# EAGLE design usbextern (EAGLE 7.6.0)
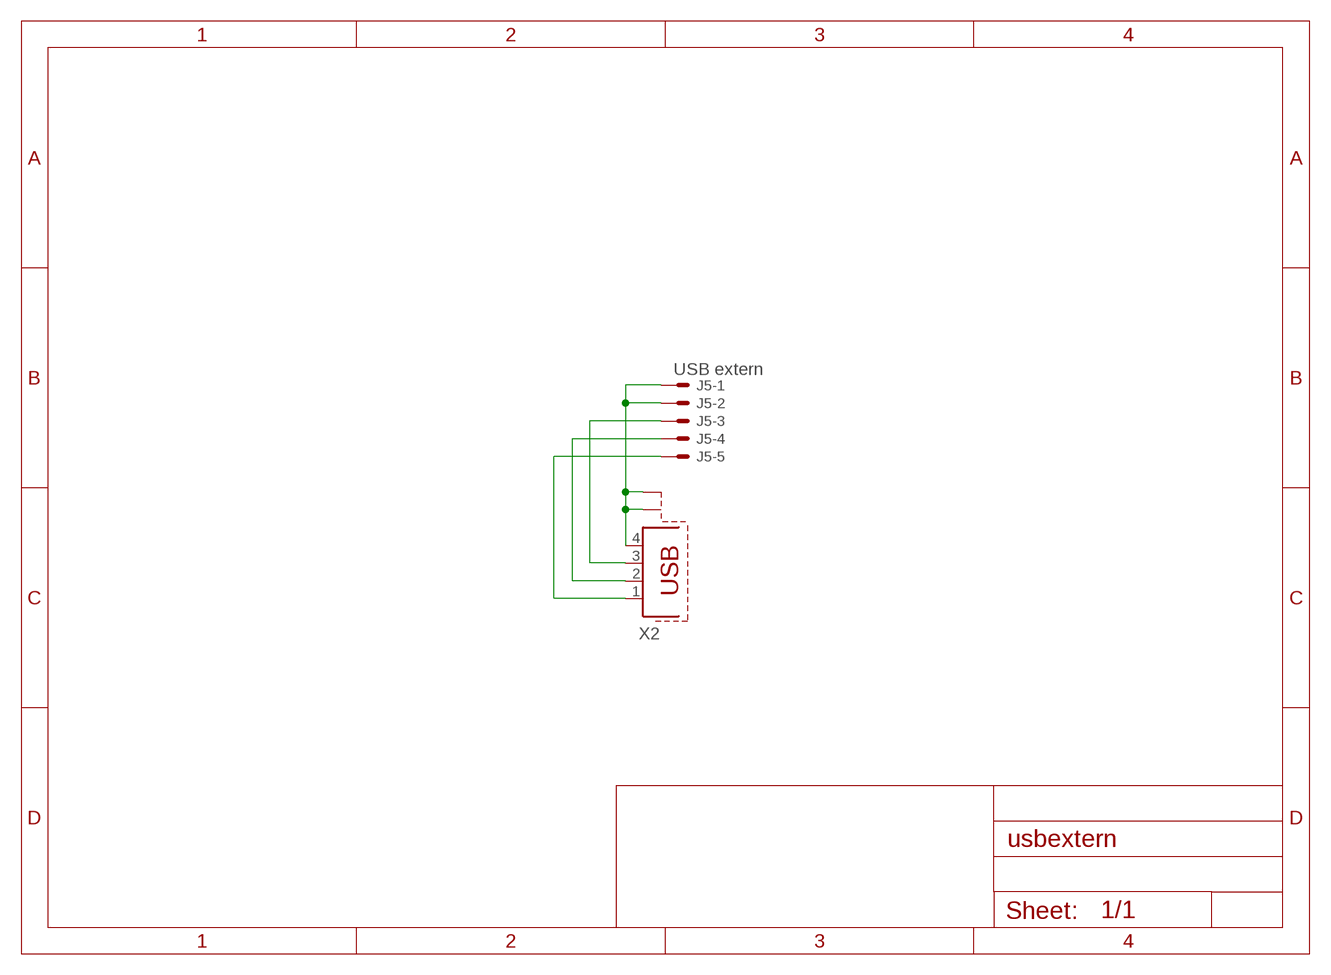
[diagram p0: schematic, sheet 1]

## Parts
J5  USB extern  22-27-2051-05  [6410-05]
X2  ev. nicht bestücken  PN61729-S  [PN61729-S]

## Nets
GND: J5.1 J5.2 X2.4 X2.S1 X2.S2
N$11: J5.5 X2.1
N$68: J5.3 X2.3
N$69: J5.4 X2.2

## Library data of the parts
J5 = con-molex:22-?-05: CONNECTOR wire to board 2.54 mm (.1 inch) pitch header; OC_FARNELL: unknown; OC_NEWARK: unknown
X2 = con-berg:PN61729-S: BERG USB connector

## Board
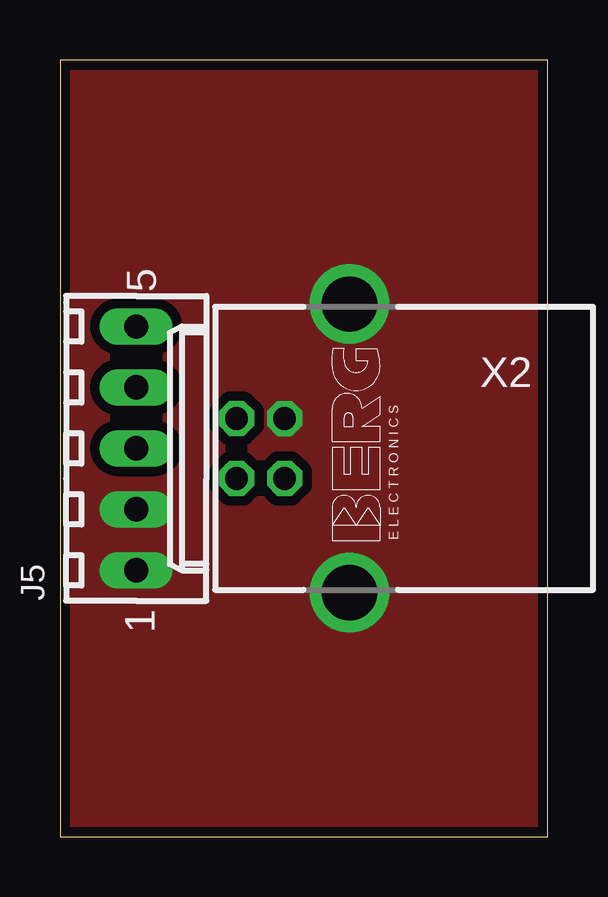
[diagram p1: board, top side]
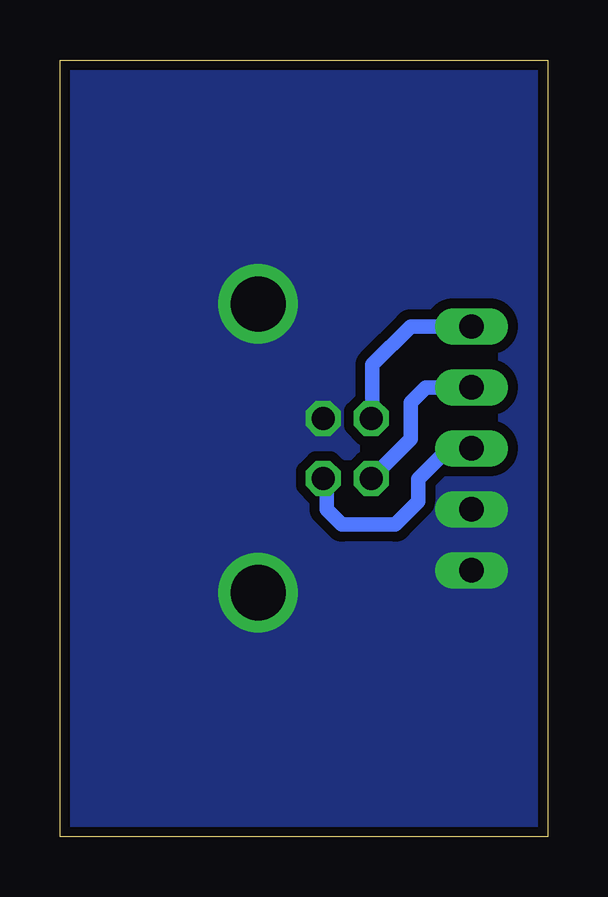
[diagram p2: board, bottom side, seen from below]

Size 20.32 x 32.38 mm. Coordinates in mm from the lower left corner, seen from the top.
Outline: 0,32.38 0,0 20.32,0 20.32,32.38 0,32.38
Copper layers (1*16): Top 0.035mm / dielectric 1.5mm / Bottom 0.035mm
Design rules "default *": minimum track width 10mil, minimum drill 24mil, track to track 8mil, track to pad 8mil, pad to pad 8mil, via to via 8mil, smd to smd 8mil, copper to edge 1mil, drill to drill 8mil, minimum pad ring 10mil, minimum via ring 8mil, stop-mask expansion 4mil, vias tented up to drill 0mil, thermal gap 10mil

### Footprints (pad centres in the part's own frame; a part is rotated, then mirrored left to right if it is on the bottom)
6410-05 = drill 1.016 long: 1 5.08,0; 2 2.54,0; 3 0,0; 4 -2.54,0; 5 -5.08,0
PN61729-S = drill 0.95 octagon: 1 1.25,4.71; 2 -1.25,4.71; 3 -1.25,2.71; 4 1.25,2.71 | drill 2.3 pad 2.9: S1 -6.02,0; S2 6.02,0

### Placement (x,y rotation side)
J5  3.17,16.19 270 top
X2  12.06,16.19 90 top

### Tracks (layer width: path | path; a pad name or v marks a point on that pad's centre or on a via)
GND
  pour Bottom (isolate 0.406, no thermals): 0,0 20.32,0 20.32,32.38 0,32.38
  pour Top (isolate 0.406, no thermals): 0,0 20.32,0 20.32,32.38 0,32.38
N$11
  Bottom 0.61: J5.5 5.71,21.27 7.3,19.68 7.3,17.5 X2.1
N$68
  Bottom 0.61: J5.3 4.13,16.19 5.4,14.92 5.4,13.97 6.35,13.02 8.57,13.02 9.21,13.65 9.21,14.79 X2.3
N$69
  Bottom 0.61: J5.4 5.08,18.73 5.71,18.1 5.71,16.58 X2.2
